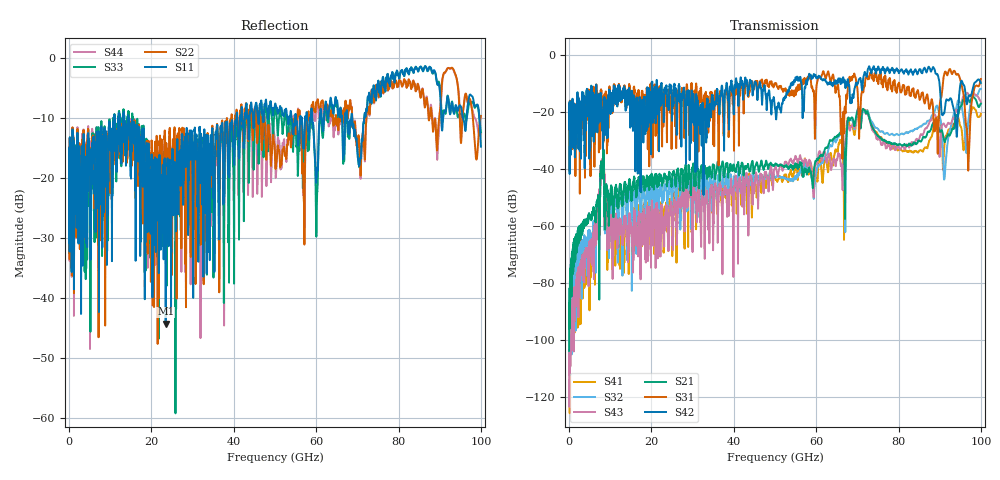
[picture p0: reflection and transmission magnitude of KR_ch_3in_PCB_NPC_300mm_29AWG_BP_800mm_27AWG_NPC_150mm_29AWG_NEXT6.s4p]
# GHz S RI R 45
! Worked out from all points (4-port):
!   4000 points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, 25 MHz to 100 GHz, reference 45 ohm
!   strongest paths, dB at 25 MHz, 25.02 GHz, 50.02 GHz, 75.03 GHz, 100 GHz:
!     S42: -21.2, -20.7, -18.6, -4.1, -9.8
!     S31: -21.2, -15.8, -10.2, -9.6, -8.4
!     S21: -103.8, -43.1, -38.3, -28.3, -17.0
!     S43: -123.3, -59.8, -39.4, -29.6, -16.4
!     S32: -108.7, -52.4, -42.9, -25.8, -11.9
!     S41: -111.6, -69.5, -43.0, -28.0, -20.5
!   lowest |S11| = -44.3 dB at 23.48 GHz (marker M1), VSWR 1.01, Z = 44.5 - j0.176 ohm
!   |S11| at or under -10 dB: start of sweep to 10.94 GHz; 14.45 GHz to 40.65 GHz (26.19 GHz wide, 95.1 % of centre); 68.74 GHz to 71.68 GHz (2.94 GHz wide, 4.19 % of centre)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
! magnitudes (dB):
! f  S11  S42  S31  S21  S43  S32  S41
! 25 MHz  -16.6  -21.2  -21.2  -103.8  -123.3  -108.7  -111.6
! 8.1 GHz  -18.4  -19.4  -21.3  -43.3  -40.9  -42.3  -40.6
! 10.88 GHz  -10.2  -10.6  -10.3  -52.5  -57.2  -57.1  -58.6
! 23.48 GHz  -44.3  -11.9  -15.8  -42.8  -56.5  -46.6  -53.4
! 91.25 GHz  -8.8  -18.6  -6.0  -30.4  -24.8  -42.1  -30.2
! 96.85 GHz  -7.7  -15.2  -36.6  -15.2  -13.4  -24.4  -23.9
! 100 GHz  -14.8  -9.8  -8.4  -17.0  -16.4  -11.9  -20.5
